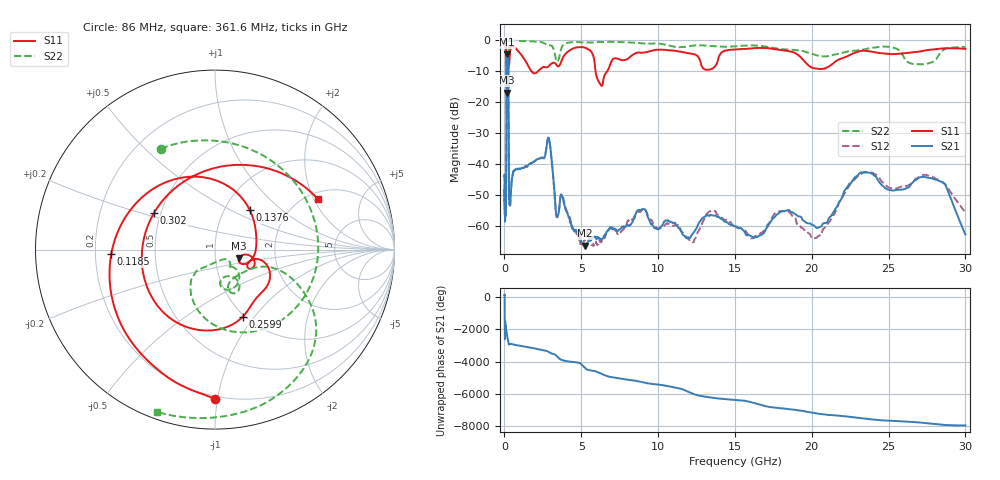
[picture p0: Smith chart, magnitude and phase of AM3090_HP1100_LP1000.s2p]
! Date/Time: Thu, Feb 28, 2019 2:06 PM
! Network Analyzer: Agilent Technologies E8364B Rev: A.07.50.67
! Sweep from 0.010 to 30.000 GHz, 1601 Points, Sweep Type: LOG
! Power Supply: 5.022 V, 0.002 A
# Hz S DB R 50
!freq MagS11 AngS11 MagS21 AngS21 MagS12 AngS12 MagS22 AngS22
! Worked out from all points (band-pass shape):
!   1601 points, 10 MHz to 30 GHz, reference 50 ohm
!   highest |S21| = -4.57 dB at 182.2 MHz (marker M1); lowest = -66.4 dB at 5.258 GHz (marker M2)
!   |S21| within 3 dB of the highest: 142.2 MHz to 244 MHz (101.8 MHz wide, 52.7 % of centre)
!   lowest |S11| = -17.0 dB at 166.5 MHz (marker M3), VSWR 1.33, Z = 65 - j6.52 ohm
!   |S11| at or under -10 dB: 136.1 MHz to 225.2 MHz (89.09 MHz wide, 49.3 % of centre); 1.746 GHz to 2.193 GHz (447.1 MHz wide, 22.7 % of centre); 5.926 GHz to 6.697 GHz (771.3 MHz wide, 12.2 % of centre)
!   |S22| runs from -23.6 to -0.1 dB; largest |S21 - S12| = 0.011
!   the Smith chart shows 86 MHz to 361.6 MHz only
!   S11 on the Smith chart (normalised r, x): 86 MHz: 0.18, -0.98; 118.5 MHz: 0.27, -0.02; 137.6 MHz: 1.31, +0.63; 259.9 MHz: 0.98, -0.88; 302 MHz: 0.46, +0.22; 361.6 MHz: 2.26, +2.15
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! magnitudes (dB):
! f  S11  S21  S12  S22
! 10 MHz  -0.3  -43.9  -44.4  -0.6
! 38.04 MHz  -0.4  -57.4  -56.1  -1.3
! 86 MHz  -1.6  -53.9  -55.7  -3.9
! 107.2 MHz  -3.3  -52.4  -52.4  -4.8
! 118.5 MHz  -4.7  -37.5  -37.5  -5.0
! 137.6 MHz  -10.7  -10.0  -9.9  -21.1
! 144.7 MHz  -12.5  -6.8  -6.8  -22.8
! 166.5 MHz  -17.0  -4.7  -4.7  -16.8
! 182.2 MHz  -13.2  -4.6  -4.6  -12.8
! 259.9 MHz  -7.8  -13.8  -13.8  -10.5
! 302 MHz  -8.0  -50.3  -49.0  -0.9
! 361.6 MHz  -3.9  -53.2  -53.4  -0.4
! 550.5 MHz  -2.0  -43.2  -43.1  -0.2
! 2.084 GHz  -10.6  -38.8  -38.8  -0.5
! 2.884 GHz  -8.4  -31.7  -31.7  -1.8
! 3.402 GHz  -8.1  -57.0  -57.3  -6.9
! 5.258 GHz  -2.5  -66.4  -64.7  -0.8
! 6.202 GHz  -14.0  -64.2  -64.7  -0.6
! 7.926 GHz  -6.3  -60.1  -59.9  -0.7
! 20.2 GHz  -9.1  -60.2  -64.1  -4.8
! 23.48 GHz  -3.5  -42.8  -42.6  -2.9
! 30 GHz  -2.8  -62.9  -55.7  -2.2
